{attribute 'qualified_only'}
{attribute 'strict'}
TYPE E_SentFastChnConfig :
(
	eValue_MsgCnt_InvMSB := 1,		// Status (1 Nibble) + Value_1 (3 Nibble) + Messagecounter (2 Nibble) + invers MSB-Value (1 Nibble) + CRC (1 Nibble)
	eValue_MsgCnt_Zero,				// Status (1 Nibble) + Value_1 (3 Nibble) + Messagecounter (2 Nibble) + Zeros (1 Nibble) + CRC (1 Nibble)
	eValue_Value,					// Status (1 Nibble) + Value_1 (3 Nibble) + Value_2 (3 Nibble) + CRC (1 Nibble)
	eValueCompact,					// Status (1 Nibble) + Value_1 (3 Nibble) + CRC (1 Nibble)
	eValueExtendet					// Status (1 Nibble) + Value_1 (4 3bit-Nibble) + CRC (1 Nibble)
);
END_TYPE
